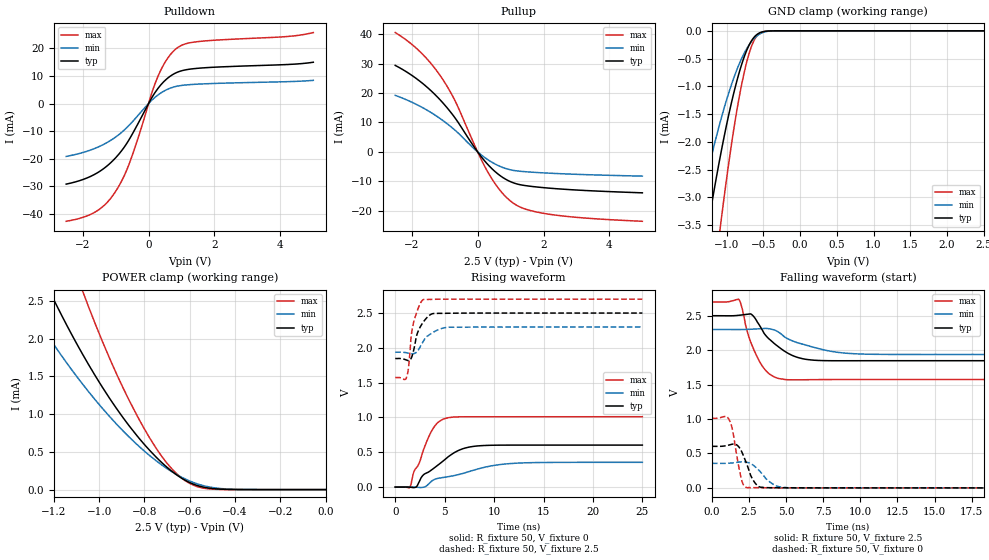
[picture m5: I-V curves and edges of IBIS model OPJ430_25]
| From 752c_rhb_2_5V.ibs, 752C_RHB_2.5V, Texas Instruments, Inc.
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[Model]   OPJ430_25
Model_type  3-state
Enable   Active-Low
Vref =   1.25
Rref =   50
Cref =   15p
Vmeas =   1.25
| variable   typ   min   max
C_comp   0.51pF   0.44pF   0.55pF
| C_pullup   1.68pF   0.43pF   2.61pF
| C_pulldown   1.48pF   0.59pF   2.43pF
| C_tri-state   0.51pF   0.44pF   0.55pF
[Temperature Range]   40   125   -40
| Ambient temperature   25   110   -40
[Voltage range]   2.5   2.3   2.7
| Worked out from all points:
|   slope of the pulldown table from 0 to 0.375 V, typ, clamps not added: 55.2 ohm
|   slope of the pullup table from 0 to 0.375 V, typ, clamps not added: 74 ohm
|   GND clamp passes 1 mA (typ) near -0.88 V on its own axis
|   POWER clamp passes 1 mA (typ) near -0.91 V on its own axis
|   rising waveform, R_fixture 50, V_fixture 0: 20-80 % time 3.27ns typ, 5.47ns min, 1.84ns max; typ from 0 V to 0.603 V
|   falling waveform, R_fixture 50, V_fixture 2.5: 20-80 % time 1.77ns typ, 2.72ns min, 1.14ns max; typ from 2.5 V to 1.85 V
|   rising waveform, R_fixture 50, V_fixture 2.5: 20-80 % time 951ps typ, 1.39ns min, 687ps max; typ from 1.85 V to 2.5 V
|   falling waveform, R_fixture 50, V_fixture 0: 20-80 % time 663ps typ, 972ps min, 493ps max; typ from 0.603 V to 0 V
[GND Clamp]
| OPJ430_25
|   Voltage   I(typ)   I(min)   I(max)
-2.5V     -16.81mA   -12.14mA   -24.1mA
-1.425V   -4.992mA   -3.561mA   -7.606mA
-1.395V   -4.723mA   -3.37mA    -7.213mA
-1.24V    -3.413mA   -2.446mA   -5.276mA
-1.08V    -2.218mA   -1.608mA   -3.473mA
-920mV    -1.216mA   -914.9uA   -1.925mA
-790mV    -584.2uA   -483.5uA   -934.3uA
-725mV    -347.7uA   -319.7uA   -555.7uA
-665mV    -187.9uA   -200.9uA   -293uA
-555mV    -39.56uA   -62.06uA   -50.17uA
-340mV    -437.8nA   -946.2nA   -241.9nA
2.5V      72.52pA    30.78nA    52.72pA
[POWER Clamp]
| OPJ430_25
|   Voltage   I(typ)   I(min)   I(max)
-2.5V     14.6mA     10.58mA    21.06mA
-1.335V   3.388mA    2.549mA    5.047mA
-1.2V     2.515mA    1.921mA    3.728mA
-1.075V   1.804mA    1.405mA    2.647mA
-1.045V   1.648mA    1.291mA    2.409mA
-925mV    1.082mA    873.8uA    1.545mA
-820mV    667.1uA    562.5uA    910.3uA
-725mV    362.2uA    330uA      446.7uA
-635mV    149.7uA    162.3uA    150.7uA
-585mV    73.88uA    95.4uA     59.77uA
-515mV    19.53uA    35.54uA    9.64uA
-31.11fV  72.52pA    293.6pA    59.75pA
[Pulldown]
| OPJ430_25
|   Voltage   I(typ)   I(min)   I(max)
-2.5V     -29.18mA   -19.14mA   -42.63mA
-1.59V    -25.33mA   -16.04mA   -39.07mA
-1.275V   -22.74mA   -14.21mA   -36.02mA
-990mV    -19.52mA   -12.05mA   -31.63mA
-760mV    -16.15mA   -9.831mA   -26.67mA
-555mV    -12.34mA   -7.425mA   -20.77mA
100mV     2.15mA     1.22mA     3.901mA
285mV     5.465mA    3.101mA    9.823mA
560mV     9.001mA    5.082mA    16.06mA
855mV     11.25mA    6.26mA     20.03mA
1.49V     12.77mA    7.029mA    22.43mA
5V        14.96mA    8.404mA    25.71mA
[Pullup]
| OPJ430_25
|   Voltage   I(typ)   I(min)   I(max)
-2.5V     29.41mA    19.22mA    40.58mA
-1.755V   24.05mA    15.55mA    34.15mA
-1.425V   20.9mA     13.45mA    30.19mA
-1.12V    17.47mA    11.19mA    25.69mA
-675mV    11.39mA    7.266mA    17.15mA
15mV      -232.4uA   -144.5uA   -367.9uA
300mV     -4.176mA   -2.587mA   -6.668mA
665mV     -7.939mA   -4.866mA   -12.86mA
1.035V    -10.32mA   -6.201mA   -17.06mA
1.455V    -11.49mA   -6.763mA   -19.48mA
2.19V     -12.36mA   -7.263mA   -21.25mA
5V        -13.94mA   -8.259mA   -23.63mA
[Ramp]
| OPJ430_25
| variable   typ   min   max
dV/dt_r   0.37/3.28E-09   0.22/5.48E-09   0.61/1.87E-09
dV/dt_f   0.41/1.81E-09   0.23/2.78E-09   0.70/1.17E-09
R_load = 50
[Rising Waveform]
| OPJ430_25
R_fixture =   50
C_fixture =   0
L_fixture =   0
V_fixture =   0
V_fixture_min = 0
V_fixture_max = 0
|   Time   V(typ)   V(min)   V(max)
0s        -6.305uV   -9.393uV   -2.931uV
1.465ns   -1.332mV   589.5uV    -5.805mV
2.12ns    83.01uV    -1.873mV   275mV
2.77ns    163.5mV    -4.057mV   497.9mV
3.61ns    240mV      76.19mV    787.4mV
5.18ns    414.3mV    145.4mV    990.3mV
6.74ns    545.9mV    191.9mV    1.01V
8.67ns    594.9mV    271.8mV    1.01V
12.91ns   603.3mV    347.5mV    1.01V
24.99ns   603.3mV    355.9mV    1.01V
[Falling Waveform]
| OPJ430_25
R_fixture =   50
C_fixture =   0
L_fixture =   0
V_fixture =   2.5
V_fixture_min = 2.3
V_fixture_max = 2.7
|   Time   V(typ)   V(min)   V(max)
0s        2.5V       2.3V       2.7V
1.805ns   2.506V     2.299V     2.74V
1.995ns   2.511V     2.3V       2.639V
2.5ns     2.524V     2.303V     2.186V
3.105ns   2.393V     2.309V     1.878V
3.755ns   2.182V     2.314V     1.676V
4.535ns   2.04V      2.255V     1.587V
6.2ns     1.872V     2.082V     1.57V
9.155ns   1.846V     1.954V     1.573V
24.99ns   1.847V     1.937V     1.573V
[Rising Waveform]
| OPJ430_25
R_fixture =   50
C_fixture =   0
L_fixture =   0
V_fixture =   2.5
V_fixture_min = 2.3
V_fixture_max = 2.7
|   Time   V(typ)   V(min)   V(max)
0s        1.847V     1.937V     1.573V
1.135ns   1.826V     1.93V      1.572V
1.34ns    1.817V     1.924V     1.712V
1.595ns   1.844V     1.917V     2.139V
1.795ns   1.927V     1.915V     2.325V
2.23ns    2.206V     1.949V     2.532V
2.885ns   2.38V      2.105V     2.695V
3.735ns   2.489V     2.214V     2.696V
5.385ns   2.497V     2.296V     2.7V
24.99ns   2.5V       2.3V       2.7V
[Falling Waveform]
| OPJ430_25
R_fixture =   50
C_fixture =   0
L_fixture =   0
V_fixture =   0
V_fixture_min = 0
V_fixture_max = 0
|   Time   V(typ)   V(min)   V(max)
0s        603.1mV    355.8mV    1.01V
1.175ns   623.2mV    358.6mV    983.1mV
1.395ns   635.1mV    362.7mV    830.5mV
2.025ns   516.6mV    377.9mV    96.36mV
2.37ns    332.3mV    371.4mV    1.88mV
2.69ns    146.3mV    342.4mV    3.284mV
3.125ns   23.39mV    263.7mV    2.486mV
3.935ns   2.144mV    79.95mV    648.5uV
4.75ns    1.829mV    7.303mV    33.06uV
24.99ns   217.1nV    153.5nV    75.54nV
